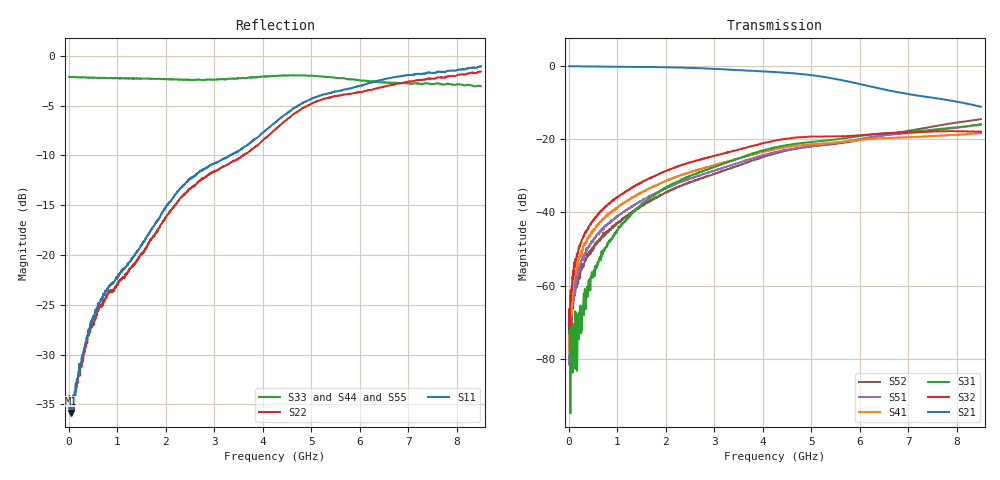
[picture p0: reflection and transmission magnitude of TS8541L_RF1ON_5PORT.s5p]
! Created with skrf (http://scikit-rf.org).
# Hz S RI R 50.0
!freq ReS11 ImS11 ReS12 ImS12 ReS13 ImS13
! ReS14 ImS14 ReS15 ImS15
! ReS21 ImS21 ReS22 ImS22 ReS23 ImS23
! ReS24 ImS24 ReS25 ImS25
! ReS31 ImS31 ReS32 ImS32 ReS33 ImS33
! ReS34 ImS34 ReS35 ImS35
! ReS41 ImS41 ReS42 ImS42 ReS43 ImS43
! ReS44 ImS44 ReS45 ImS45
! ReS51 ImS51 ReS52 ImS52 ReS53 ImS53
! ReS54 ImS54 ReS55 ImS55
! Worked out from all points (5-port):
!   1601 points, 10 MHz to 8.5 GHz, reference 50 ohm
!   strongest paths, dB at 10 MHz, 2.132 GHz, 4.255 GHz, 6.378 GHz, 8.5 GHz:
!     S21: -0.1, -0.5, -1.7, -6.1, -11.2
!     S32: -71.7, -28.1, -20.4, -18.6, -18.0
!     S31: -70.7, -32.3, -22.3, -18.6, -16.1
!     S41: -77.5, -30.7, -22.8, -19.8, -18.4
!     S51: -81.6, -32.7, -23.6, -19.2, -15.9
!     S52: -76.2, -33.8, -23.9, -19.2, -14.6
!   lowest |S11| = -35.8 dB at 47.14 MHz (marker M1), VSWR 1.03, Z = 51.6 - j0.343 ohm
!   |S11| at or under -10 dB: start of sweep to 3.328 GHz
